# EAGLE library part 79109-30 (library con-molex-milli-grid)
RECEPTACAL
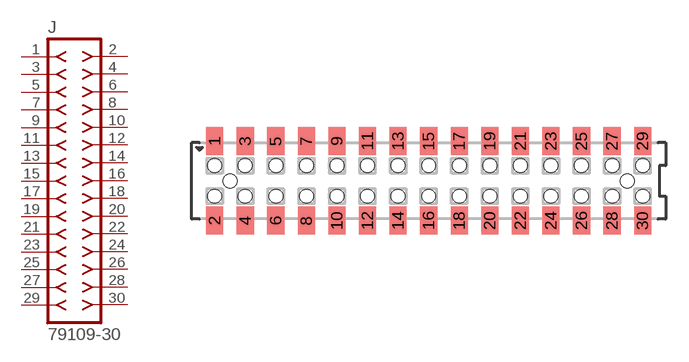
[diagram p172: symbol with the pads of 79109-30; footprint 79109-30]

Designator prefix J

## 79109-30  [79109-30]
1  1  pas
2  2  pas
3  3  pas
4  4  pas
5  5  pas
6  6  pas
7  7  pas
8  8  pas
9  9  pas
10  10  pas
11  11  pas
12  12  pas
13  13  pas
14  14  pas
15  15  pas
16  16  pas
17  17  pas
18  18  pas
19  19  pas
20  20  pas
21  21  pas
22  22  pas
23  23  pas
24  24  pas
25  25  pas
26  26  pas
27  27  pas
28  28  pas
29  29  pas
30  30  pas

## Footprint 79109-30 (pad centres in mm)
RECEPTACAL SMD Dual Row, Vertical, Pass-Thru
smd 1.12 x 1.83: 1 -14,2.6; 2 -14,-2.6; 3 -12,2.6; 4 -12,-2.6; 5 -10,2.6; 6 -10,-2.6; 7 -8,2.6; 8 -8,-2.6; 9 -6,2.6; 10 -6,-2.6; 11 -4,2.6; 12 -4,-2.6; 13 -2,2.6; 14 -2,-2.6; 15 0,2.6; 16 0,-2.6; 17 2,2.6; 18 2,-2.6; 19 4,2.6; 20 4,-2.6; 21 6,2.6; 22 6,-2.6; 23 8,2.6; 24 8,-2.6; 25 10,2.6; 26 10,-2.6; 27 12,2.6; 28 12,-2.6; 29 14,2.6; 30 14,-2.6
hole 0.914 at -13,0
hole 0.914 at -14,1
hole 0.914 at -14,-1
hole 0.914 at -12,-1
hole 0.914 at -12,1
hole 0.914 at -10,-1
hole 0.914 at -10,1
hole 0.914 at 13,0
hole 0.914 at -8,1
hole 0.914 at -8,-1
hole 0.914 at -6,1
hole 0.914 at -6,-1
hole 0.914 at -4,1
hole 0.914 at -4,-1
hole 0.914 at -2,1
hole 0.914 at -2,-1
hole 0.914 at 0,-1
hole 0.914 at 0,1
hole 0.914 at 2,1
hole 0.914 at 2,-1
hole 0.914 at 4,1
hole 0.914 at 4,-1
hole 0.914 at 6,1
hole 0.914 at 6,-1
hole 0.914 at 8,-1
hole 0.914 at 8,1
hole 0.914 at 10,1
hole 0.914 at 12,1
hole 0.914 at 14,1
hole 0.914 at 10,-1
hole 0.914 at 12,-1
hole 0.914 at 14,-1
